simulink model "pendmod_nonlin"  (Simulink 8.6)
settings: Solver=ode45  StartTime=0.0  StopTime=100  RelTol=1e-3
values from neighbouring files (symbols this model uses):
  g = 9.81    [test_omega.m]
  I = 0.03159    [test_omega.m]
  L = length(teta)-1    [fft_teta.m]
  m = 0.23    [test_omega.m]
undefined symbols (not defined in the file or in its folder): cart_friction, cM, d, J, Kb, Kt, magnitude, pend_damp, R, theta0

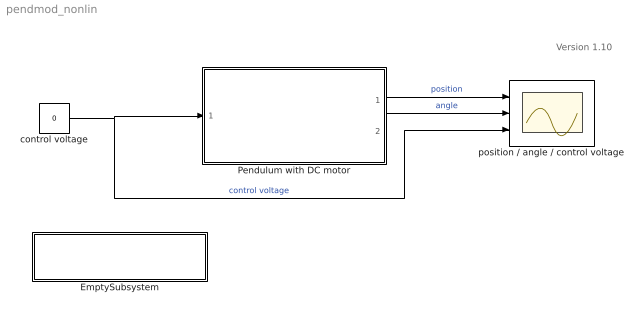
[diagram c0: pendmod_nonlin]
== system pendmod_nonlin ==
  note: Version 1.10
  EmptySubsystem : Subsystem
  Pendulum with DC motor : Subsystem
  control voltage : Constant  Value=0
  position / angle / control voltage : Scope  NumInputPorts=3
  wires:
  Pendulum with DC motor/1(x) -> position / angle / control voltage/1  "position"
  Pendulum with DC motor/2(theta) -> position / angle / control voltage/2  "angle"
  control voltage/1 -> position / angle / control voltage/3, Pendulum with DC motor/1(v)  "control voltage"

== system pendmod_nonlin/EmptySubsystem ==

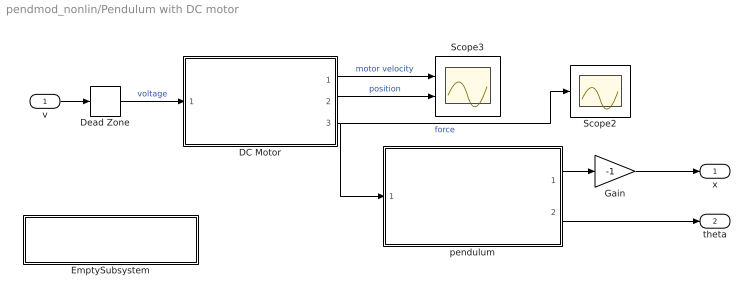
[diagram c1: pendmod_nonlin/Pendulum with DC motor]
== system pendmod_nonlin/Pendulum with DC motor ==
  v : Inport
  DC Motor : Subsystem
  Dead Zone : DeadZone  LowerValue=-0.05  UpperValue=0.05
  EmptySubsystem : Subsystem
  Gain : Gain  Gain=-1
  Scope2 : Scope
  Scope3 : Scope  NumInputPorts=2
  pendulum : Subsystem
  x : Outport
  theta : Outport  Port=2
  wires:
  Dead Zone/1 -> DC Motor/1(voltage)  "voltage"
  Gain/1 -> x/1
  pendulum/2(pendulum angle in radians) -> theta/1
  pendulum/1(cart possition) -> Gain/1
  v/1 -> Dead Zone/1
  DC Motor/1(motor velocity) -> Scope3/1  "motor velocity"
  DC Motor/2(motor position - radians) -> Scope3/2  "position"
  DC Motor/3(force) -> pendulum/1(driving force F), Scope2/1  "force"

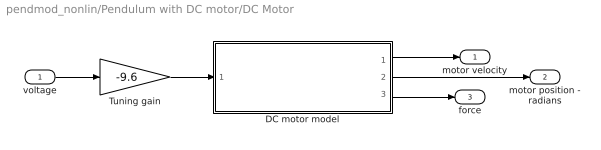
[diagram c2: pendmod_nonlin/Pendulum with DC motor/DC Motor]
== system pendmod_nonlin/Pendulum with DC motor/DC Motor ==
  voltage : Inport
  DC motor model : Subsystem
  Tuning gain : Gain  Gain=-9.6
  motor velocity : Outport
  motor position - radians : Outport  Port=2
  force : Outport  Port=3
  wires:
  DC motor model/3(force) -> force/1
  DC motor model/1(motor velocity) -> motor velocity/1
  voltage/1 -> Tuning gain/1
  DC motor model/2(motor position -radians) -> motor position - radians/1
  Tuning gain/1 -> DC motor model/1(control voltage)

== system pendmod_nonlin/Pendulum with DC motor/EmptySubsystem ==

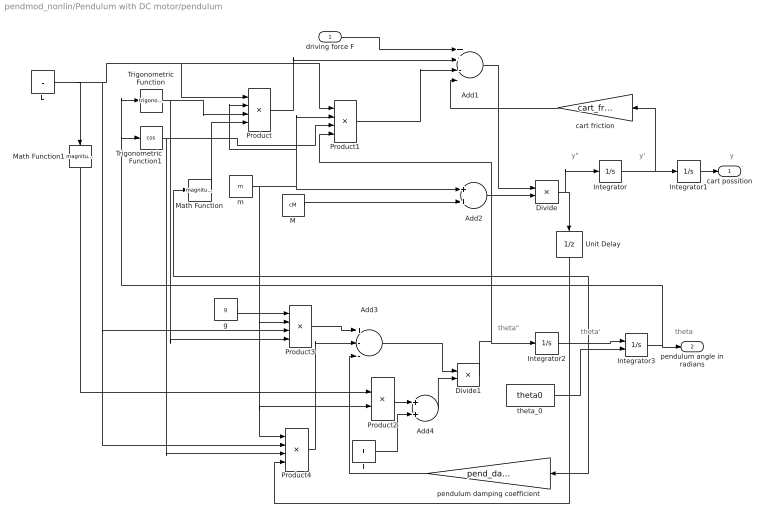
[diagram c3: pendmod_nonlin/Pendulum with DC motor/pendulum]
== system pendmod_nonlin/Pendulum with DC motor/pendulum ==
  note: y"
  note: y'
  note: theta"
  note: theta'
  note: theta
  note: y
  driving force F : Inport
  Add1 : Sum  Inputs=++--
  Add2 : Sum
  Add3 : Sum  Inputs=+--
  Add4 : Sum
  Divide : Product  Inputs=*/
  Divide1 : Product  Inputs=*/
  I : Constant  Value=I
  Integrator : Integrator
  Integrator1 : Integrator
  Integrator2 : Integrator
  Integrator3 : Integrator  InitialConditionSource=external
  L : Constant  Value=L
  M : Constant  Value=cM
  Math Function : Math  Operator=magnitude^2
  Math Function1 : Math  Operator=magnitude^2
  Product{,1,3..4} (4 alike) : Product  Inputs=4
  Product2 : Product
  Trigonometric Function : Trigonometry
  Trigonometric Function1 : Trigonometry  Operator=cos
  Unit Delay : UnitDelay  SampleTime=0.001
  cart friction : Gain  Gain=cart_friction
  g : Constant  Value=g
  m : Constant  Value=m
  pendulum damping coefficient : Gain  Gain=pend_damp
  theta_0 : Constant  Value=theta0
  cart possition : Outport
  pendulum angle in radians : Outport  Port=2
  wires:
  Unit Delay/1 -> Product4/4
  I/1 -> Add4/2
  Add4/1 -> Divide1/2
  Product2/1 -> Add4/1
  Integrator1/1 -> cart possition/1
  driving force F/1 -> Add1/1
  pendulum damping coefficient/1 -> Add3/3
  cart friction/1 -> Add1/4
  g/1 -> Product3/1
  Product4/1 -> Add3/2
  Product3/1 -> Add3/1
  Math Function1/1 -> Product2/1
  Add3/1 -> Divide1/1
  Trigonometric Function1/1 -> Product4/3, Product1/3
  Product1/1 -> Add1/3
  Product/1 -> Add1/2
  Math Function/1 -> Product/4
  theta_0/1 -> Integrator3/2
  Trigonometric Function/1 -> Product3/4, Product/3
  L/1 -> Product4/2, Product3/3, Product1/1, Product/1, Math Function1/1
  Divide1/1 -> Product1/4, Integrator2/1
  Divide/1 -> Unit Delay/1, Integrator/1
  Add1/1 -> Divide/1
  Add2/1 -> Divide/2
  M/1 -> Add2/2
  m/1 -> Product4/1, Product2/2, Product3/2, Product1/2, Product/2, Add2/1
  Integrator3/1 -> pendulum angle in radians/1, Trigonometric Function/1, Trigonometric Function1/1
  Integrator2/1 -> pendulum damping coefficient/1, Math Function/1, Integrator3/1
  Integrator/1 -> cart friction/1, Integrator1/1

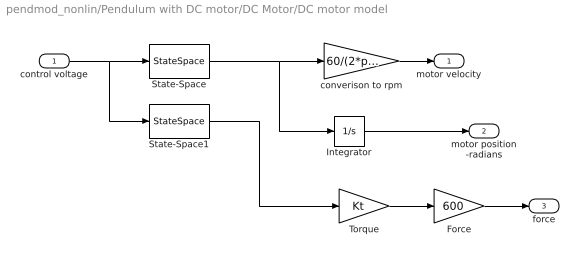
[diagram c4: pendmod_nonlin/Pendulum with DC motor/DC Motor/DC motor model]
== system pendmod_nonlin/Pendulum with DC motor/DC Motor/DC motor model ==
  control voltage : Inport
  Force : Gain  Gain=600
  Integrator : Integrator
  State-Space : StateSpace  A=[-d/J Kt/J;-Kb/L -R/L]  B=[0; 1/L]  C=[1 0]  D=0  X0=0
  State-Space1 : StateSpace  A=[-d/J Kt/J;-Kb/L -R/L]  B=[0; 1/L]  C=[0 1]  D=0  X0=0
  Torque : Gain  Gain=Kt
  converison to rpm : Gain  Gain=60/(2*pi)
  motor velocity : Outport
  motor position -radians : Outport  Port=2
  force : Outport  Port=3
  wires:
  Force/1 -> force/1
  Torque/1 -> Force/1
  State-Space1/1 -> Torque/1
  State-Space/1 -> Integrator/1, converison to rpm/1
  control voltage/1 -> State-Space1/1, State-Space/1
  Integrator/1 -> motor position -radians/1
  converison to rpm/1 -> motor velocity/1
